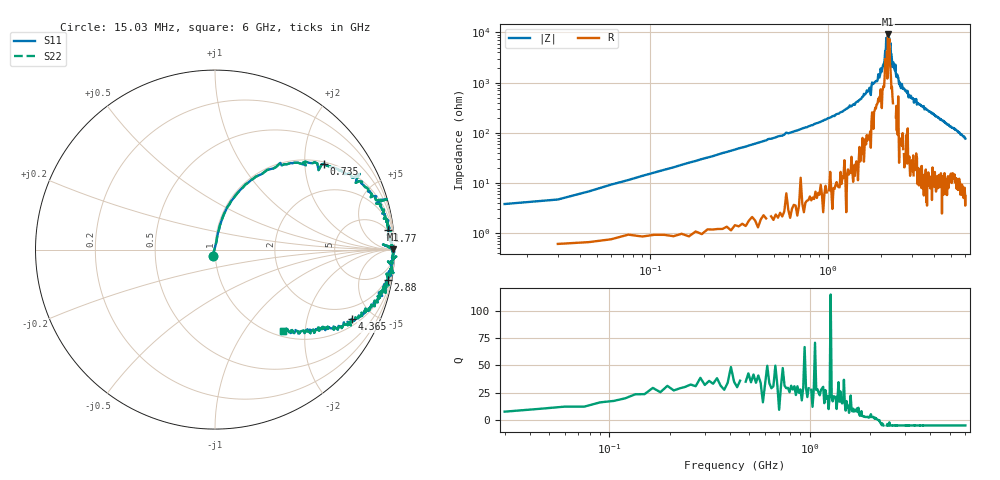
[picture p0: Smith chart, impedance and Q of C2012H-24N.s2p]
!	Network	Analyzer	HP8753E.07.74:	Oct	30	2002	Serial	No.	JP38451487
!	Hewlett-Packard
!	28	Aug	2009	9:55:31
!	Frequency	S11	S21	S12	S22
#	HZ	S	RI	R	50
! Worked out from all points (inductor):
!   400 points, 15.03 MHz to 6 GHz, reference 50 ohm
!   read as one part in series: L = 24.3 nH near 45.03 MHz
!   highest |Z| = 9.13 kohm at 2.19 GHz (marker M1)
!   self-resonance near 2.19 GHz
!   S11 on the Smith chart (normalised r, x): 15.03 MHz: 0.97, -0.07; 735 MHz: 1.05, +2.50; 1.77 GHz: 4, +17; 2.88 GHz: 2, -11; 4.365 GHz: 1.31, -3.75; 6 GHz: 1.11, -1.54
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1.502992e7  -0.0129 -0.037  1.01 0.037  1.01 0.037  -0.0129 -0.037
9.002955e7  0.027 0.134  0.973 -0.134  0.973 -0.134  0.027 0.134
1.95029e8  0.0905 0.271  0.91 -0.271  0.91 -0.271  0.0905 0.271
7.350263e8  0.607 0.478  0.393 -0.478  0.393 -0.478  0.607 0.478
1.020025e9  0.788 0.391  0.212 -0.391  0.212 -0.391  0.788 0.391
1.755021e9  0.956 0.165  0.0439 -0.165  0.0439 -0.165  0.956 0.165
1.770021e9  0.966 0.107  0.0342 -0.107  0.0342 -0.107  0.966 0.107
2.01002e9  0.979 0.0568  0.0214 -0.0568  0.0214 -0.0568  0.979 0.0568
2.130019e9  0.988 0.0214  0.0123 -0.0214  0.0123 -0.0214  0.988 0.0214
2.145019e9  1 0.0128  -0.00054 -0.0128  -0.00054 -0.0128  1 0.0128
2.160019e9  0.988 0.0119  0.0115 -0.0119  0.0115 -0.0119  0.988 0.0119
2.175019e9  0.936 0.0284  0.0641 -0.0284  0.0641 -0.0284  0.936 0.0284
2.190019e9  0.99 0.00272  0.0105 -0.00272  0.0105 -0.00272  0.99 0.00272
2.265019e9  0.995 -0.0152  0.0051 0.0152  0.0051 0.0152  0.995 -0.0152
2.325018e9  0.986 -0.0459  0.0145 0.0459  0.0145 0.0459  0.986 -0.0459
2.595017e9  0.992 -0.128  0.00809 0.128  0.00809 0.128  0.992 -0.128
2.880016e9  0.962 -0.167  0.038 0.167  0.038 0.167  0.962 -0.167
3.015015e9  0.968 -0.198  0.0324 0.198  0.0324 0.198  0.968 -0.198
4.00501e9  0.827 -0.36  0.173 0.36  0.173 0.36  0.827 -0.36
4.365008e9  0.762 -0.386  0.238 0.386  0.238 0.386  0.762 -0.386
5.010005e9  0.619 -0.438  0.381 0.438  0.381 0.438  0.619 -0.438
6e9  0.381 -0.451  0.619 0.451  0.619 0.451  0.381 -0.451
